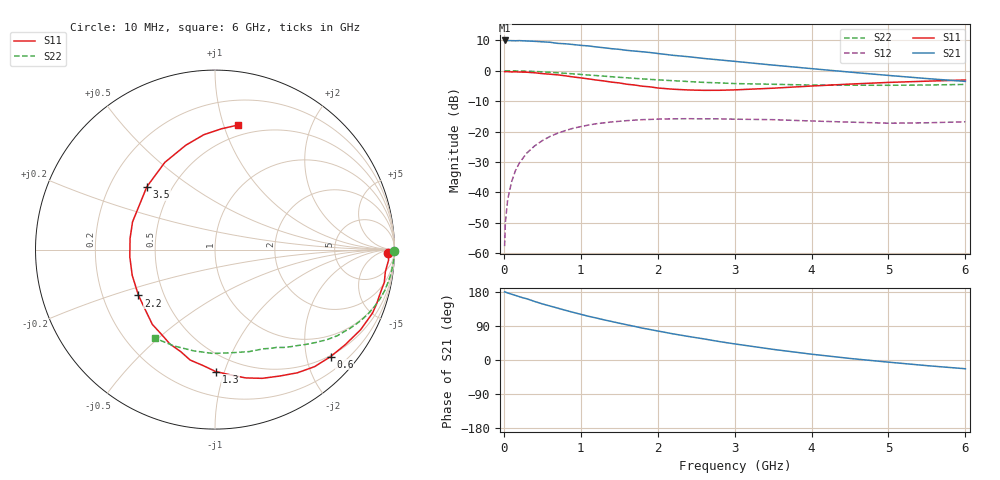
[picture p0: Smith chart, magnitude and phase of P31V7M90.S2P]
! SIEMENS Small Signal Semiconductors
! BFP181
! Si NPN RF Bipolar Junction Transistor in SOT143
! VCE = 1.75 V  IC = 0.9 mA
! Common Emitter S-Parameters:  March  1996
# GHz  S  MA  R  50
!  f  S11  S21  S12  S22
! GHz  MAG  ANG  MAG  ANG  MAG  ANG  MAG  ANG
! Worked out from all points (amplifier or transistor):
!   36 points, 10 MHz to 6 GHz, reference 50 ohm
!   highest |S21| = 10.0 dB at 10 MHz (marker M1)
!   |S21| within 3 dB of that: start of sweep to 1.523 GHz
!   unconditionally stable (mu >= 1): 3.156 GHz to end of sweep
!   at 250 MHz: K = 0.09, MSG = 19.3 dB, |S12| = -28.7 dB
!   at 1.4 GHz: K = 0.49, MSG = 12.1 dB, |S12| = -16.8 dB
!   at 6 GHz: K = 1.33, MAG = 3.2 dB, |S12| = -16.8 dB
!   S11 on the Smith chart (normalised r, x): 10 MHz: 45, -22; 600 MHz: 0.48, -2.47; 1.3 GHz: 0.37, -0.94; 2.2 GHz: 0.36, -0.24; 3.5 GHz: 0.36, +0.35; 6 GHz: 0.40, +1.12
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0.01  0.9647 -1.0  3.152 179.7  0.0013 83.9  0.9985 -0.3
0.02  0.9662 -1.6  3.132 179.4  0.0032 89.4  0.998 -0.6
0.05  0.9688 -3.5  3.142 176.9  0.0076 89.3  0.9969 -1.7
0.1  0.9572 -7.3  3.128 173.7  0.0148 86.6  0.9971 -3.4
0.15  0.9608 -11.0  3.116 170.5  0.0226 82.0  0.9936 -5.1
0.25  0.9498 -18.4  3.111 164.0  0.0367 77.8  0.9879 -8.5
0.3  0.9463 -21.9  3.089 161.5  0.0444 75.3  0.9826 -10.2
0.4  0.9258 -28.9  3.05 154.5  0.058 70.9  0.9733 -13.5
0.6  0.8777 -42.8  2.945 142.5  0.0831 61.4  0.9433 -19.7
0.8  0.8258 -56.2  2.779 131.2  0.1037 53.1  0.908 -25.3
1.1  0.7349 -76.6  2.561 115.4  0.1278 42.1  0.8511 -32.6
1.3  0.6799 -89.6  2.391 106.1  0.139 35.4  0.8154 -37.1
1.5  0.6307 -102.7  2.252 97.2  0.1474 30.1  0.78 -40.8
1.8  0.557 -122.8  2.054 84.2  0.1569 23.0  0.7361 -45.7
2.2  0.4969 -149.1  1.795 69.0  0.162 14.7  0.6862 -52.0
2.4  0.483 -162.7  1.702 62.1  0.1626 11.1  0.6649 -55.1
2.8  0.4773 172.5  1.51 48.7  0.1616 5.5  0.6313 -60.7
3.5  0.5166 137.3  1.239 28.1  0.1568 -1.6  0.5991 -71.6
4  0.5606 119.9  1.084 15.3  0.1491 -4.5  0.582 -80.9
4.5  0.6037 105.7  0.95 4.1  0.1429 -6.3  0.5787 -91.2
5.5  0.6739 87.0  0.744 -14.9  0.1393 -2.7  0.583 -112.8
6  0.7053 79.6  0.668 -23.1  0.1446 -1.4  0.5958 -123.9
